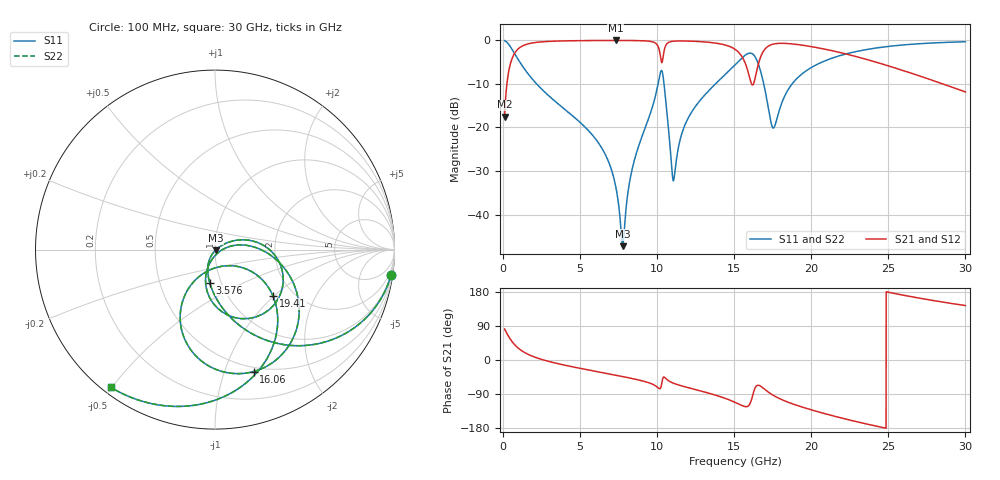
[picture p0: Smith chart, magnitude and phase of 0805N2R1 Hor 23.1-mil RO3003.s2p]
# GHz S MA R 50
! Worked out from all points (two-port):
!   3201 points, 100 MHz to 30 GHz, reference 50 ohm
!   highest |S21| = -0.04 dB at 7.313 GHz (marker M1); lowest = -17.5 dB at 100 MHz (marker M2)
!   |S21| within 3 dB of the highest: 740 MHz to 10.18 GHz (9.443 GHz wide, 173 % of centre); 16.81 GHz to 22.14 GHz (5.332 GHz wide, 27.4 % of centre)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
!   lowest |S11| = -47.2 dB at 7.762 GHz (marker M3), VSWR 1.01, Z = 50.3 - j0.303 ohm
!   |S11| at or under -10 dB: 2.176 GHz to 10.06 GHz (7.881 GHz wide, 129 % of centre); 10.44 GHz to 13.78 GHz (3.341 GHz wide, 27.6 % of centre); 16.91 GHz to 18.76 GHz (1.843 GHz wide, 10.3 % of centre)
!   |S22| runs from -47.2 to -0.1 dB; largest |S21 - S12| = 0
!   S11 on the Smith chart (normalised r, x): 100 MHz: 1, -14; 3.576 GHz: 0.88, -0.34; 16.06 GHz: 0.46, -1.26; 19.41 GHz: 1.58, -0.98; 30 GHz: 0.02, -0.50
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0.1  0.9911 -8.2  0.1329 81.8  0.1329 81.8  0.9911 -8.2
0.4270312  0.8675 -32.3  0.4971 57.7  0.4971 57.7  0.8675 -32.3
0.8755312  0.6467 -54.7  0.7619 35.2  0.7619 35.2  0.6467 -54.7
1.81925  0.3732 -78.4  0.9263 11.4  0.9263 11.4  0.3732 -78.4
3.575875  0.1865 -99.2  0.9802 -9.8  0.9802 -9.8  0.1865 -99.2
5.089563  0.1106 -111.3  0.991 -22.7  0.991 -22.7  0.1106 -111.3
6.537844  0.05287 -120.4  0.995 -34.1  0.995 -34.1  0.05287 -120.4
7.313375  0.02095 -119.4  0.9956 -40.1  0.9956 -40.1  0.02095 -119.4
7.761875  0.004356 -43.7  0.9954 -43.7  0.9954 -43.7  0.004356 -43.7
8.406594  0.03504 31.9  0.9936 -49.1  0.9936 -49.1  0.03504 31.9
10.06978  0.3248 -3.6  0.8408 -73.6  0.8408 -73.6  0.3248 -3.6
10.38747  0.3815 -76.9  0.6524 -46.3  0.6524 -46.3  0.3815 -76.9
11.07891  0.02513 -37.2  0.9767 -61.6  0.9767 -61.6  0.02513 -37.2
12.10672  0.1377 10.9  0.9781 -74.0  0.9781 -74.0  0.1377 10.9
15.05  0.5237 -28.8  0.7886 -111.6  0.7886 -111.6  0.5237 -28.8
16.05913  0.7126 -72.5  0.3409 -111.9  0.3409 -111.9  0.7126 -72.5
16.67581  0.4649 -114.2  0.6186 -68.3  0.6186 -68.3  0.4649 -114.2
17.52609  0.09871 -78.6  0.9035 -93.0  0.9035 -93.0  0.09871 -78.6
19.41353  0.4136 -38.7  0.8787 -124.3  0.8787 -124.3  0.4136 -38.7
20.03956  0.4915 -45.1  0.8438 -132.0  0.8438 -132.0  0.4915 -45.1
25.01978  0.8513 -92.4  0.5077 178.6  0.5077 178.6  0.8513 -92.4
30  0.9623 -127.1  0.2557 143.7  0.2557 143.7  0.9623 -127.1
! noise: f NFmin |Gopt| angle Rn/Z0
0.1  0.0009952  0.9404  1.433  0.003731
3.417  0.006415  0.7086  20.35  0.0042
6.743  0.01152  0.6903  38.39  0.006482
10.06  0.08101  0.9275  55.75  0.1939
13.39  0.03384  0.793  71.97  0.02225
16.7  0.1985  0.9536  87.96  0.4986
20.03  0.05542  0.8202  101.9  0.02603
23.35  0.05629  0.8033  114.5  0.01787
26.67  0.06835  0.8216  126.8  0.01672
30  0.08978  0.8537  138.9  0.01683
